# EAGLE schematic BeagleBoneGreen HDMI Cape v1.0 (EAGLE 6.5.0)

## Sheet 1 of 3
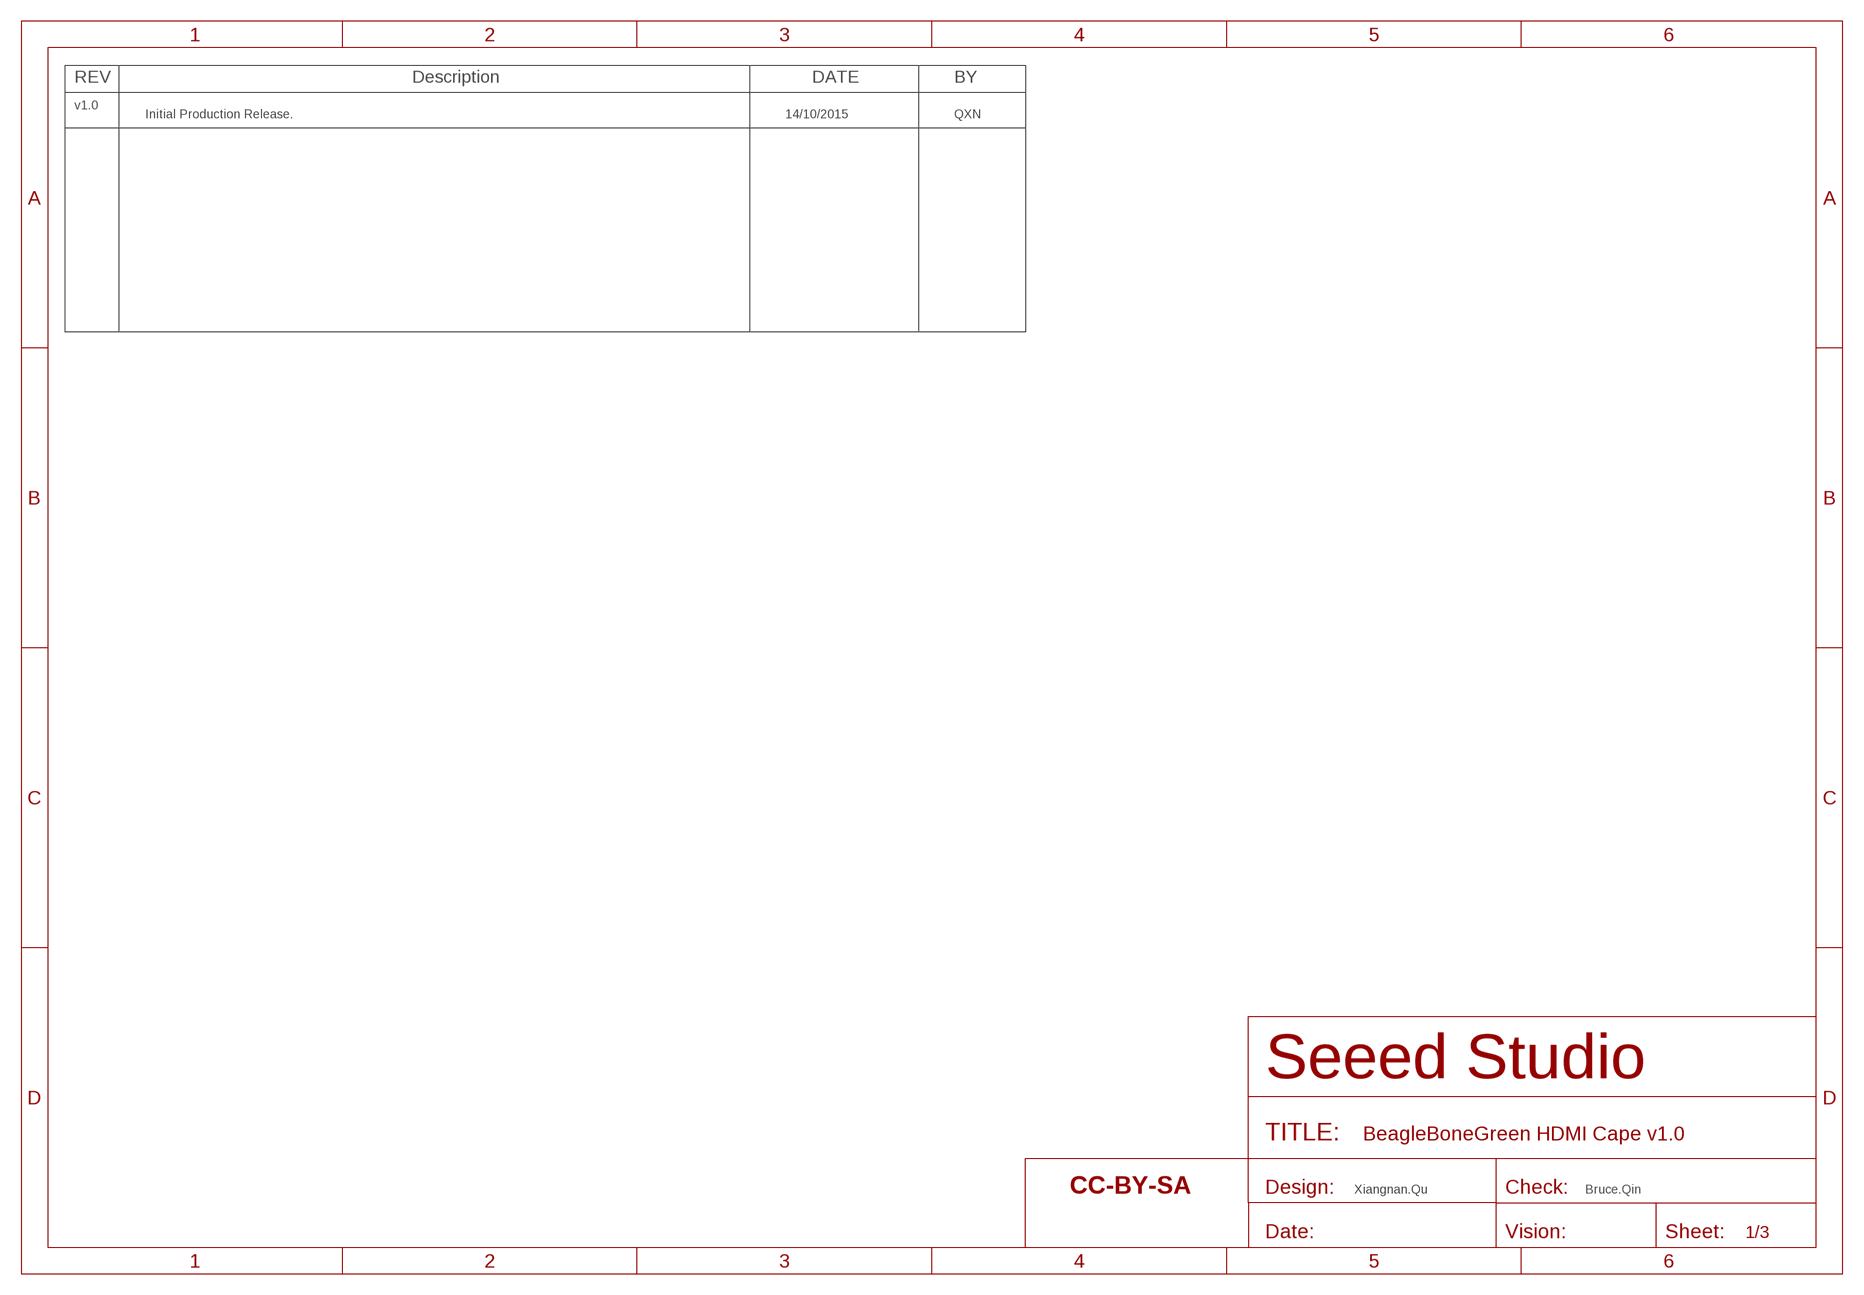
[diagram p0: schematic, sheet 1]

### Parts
FR1  SEEEDSTUDIO-OPEN-SCH-FRAME  [SEEEDSTUDIO-PCB-FRAME]

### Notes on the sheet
- REV | Description | DATE | BY
- v1.0
- Initial Production Release. | 14/10/2015 | QXN
- Xiangnan.Qu | Bruce.Qin

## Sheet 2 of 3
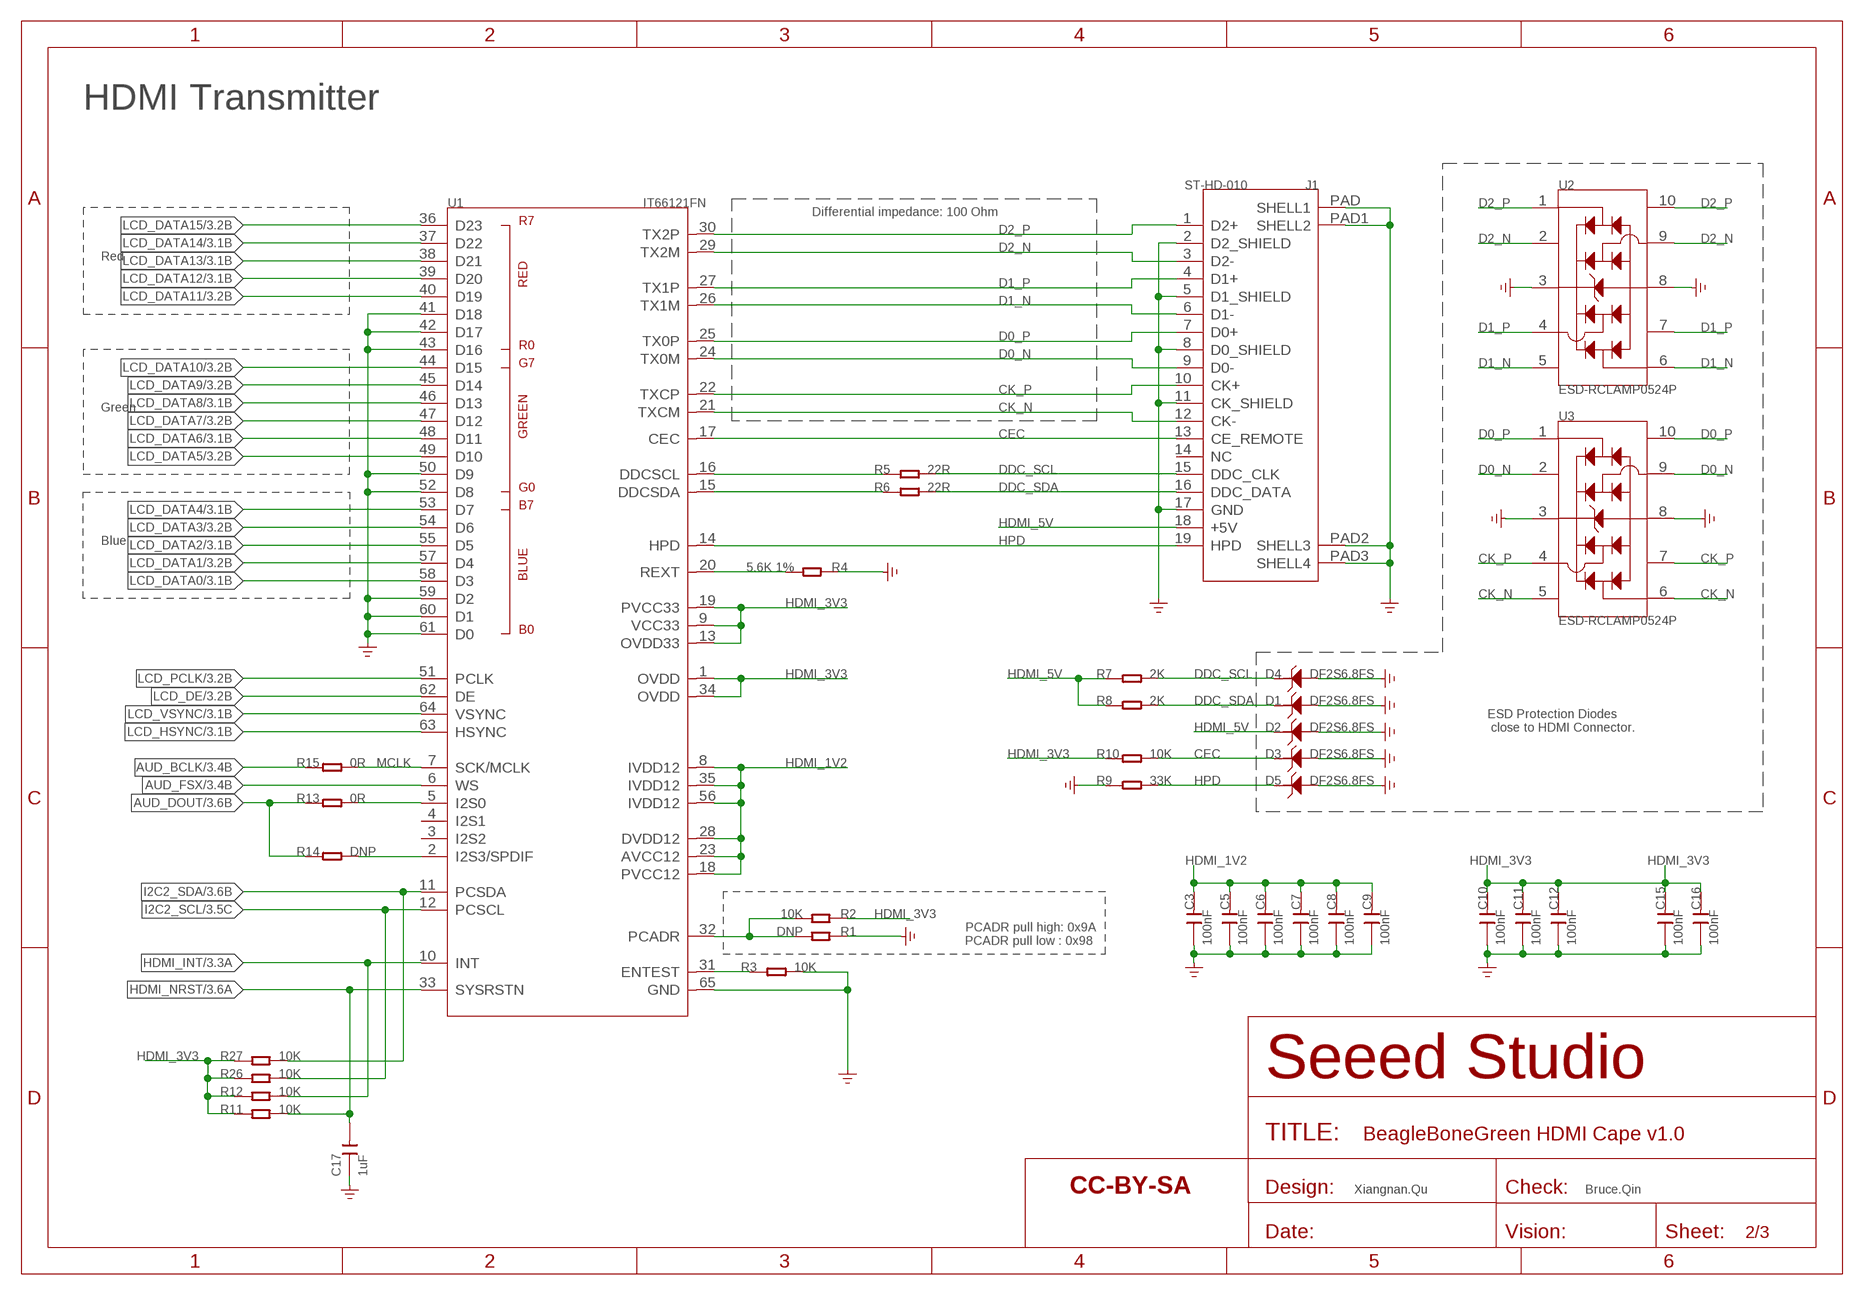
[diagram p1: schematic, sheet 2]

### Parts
C3  100nF  CAP-0402  [C0402]
C5  100nF  CAP-0402  [C0402]
C6  100nF  CAP-0402  [C0402]
C7  100nF  CAP-0402  [C0402]
C8  100nF  CAP-0402  [C0402]
C9  100nF  CAP-0402  [C0402]
C10  100nF  CAP-0402  [C0402]
C11  100nF  CAP-0402  [C0402]
C12  100nF  CAP-0402  [C0402]
C15  100nF  CAP-0402  [C0402]
C16  100nF  CAP-0402  [C0402]
C17  1uF  CAP-0603  [C0603]
D1  DF2S6.8FS  D-ESD-2P'DF2S6.8FS'  [SOD-923]
D2  DF2S6.8FS  D-ESD-2P'DF2S6.8FS'  [SOD-923]
D3  DF2S6.8FS  D-ESD-2P'DF2S6.8FS'  [SOD-923]
D4  DF2S6.8FS  D-ESD-2P'DF2S6.8FS'  [SOD-923]
D5  DF2S6.8FS  D-ESD-2P'DF2S6.8FS'  [SOD-923]
FR2  SEEEDSTUDIO-OPEN-SCH-FRAME  [SEEEDSTUDIO-PCB-FRAME]
J1  ST-HD-010  CONNECTOR-HDMI-19P  [HDMI19P-0.5-15X12.15X6.18MM]
R1  DNP  RES-0402  [R0402]
R2  10K  RES-0402  [R0402]
R3  10K  RES-0402  [R0402]
R4  5.6K 1%  RES-0402  [R0402]
R5  22R  RES-0402  [R0402]
R6  22R  RES-0402  [R0402]
R7  2K  RES-0402  [R0402]
R8  2K  RES-0402  [R0402]
R9  33K  RES-0402  [R0402]
R10  10K  RES-0402  [R0402]
R11  10K  RES-0402  [R0402]
R12  10K  RES-0402  [R0402]
R13  0R  RES-0402  [R0402]
R14  DNP  RES-0402  [R0402]
R15  0R  RES-0402  [R0402]
R26  10K  RES-0402  [R0402]
R27  10K  RES-0402  [R0402]
U1  IT66121FN  TRANSFER_IT66121FN-9  [QFN64-0.5-9X9MM]
U2  ESD-RCLAMP0524P  [ESD10P-0.5-2.5X1X0.58MM]
U3  ESD-RCLAMP0524P  [ESD10P-0.5-2.5X1X0.58MM]

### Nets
AUD_BCLK: R15.1 ; also sheet 3
AUD_DOUT: R13.1 R14.1 ; also sheet 3
AUD_FSX: U1.6(WS) ; also sheet 3
CEC: D3.1 J1.13(CE_REMOTE) R10.2 U1.17(CEC)
CK_N: J1.12(CK-) U1.21(TXCM) U3.5 U3.6
CK_P: J1.10(CK+) U1.22(TXCP) U3.4 U3.7
D0_N: J1.9(D0-) U1.24(TX0M) U3.2 U3.9
D0_P: J1.7(D0+) U1.25(TX0P) U3.1 U3.10
D1_N: J1.6(D1-) U1.26(TX1M) U2.5 U2.6
D1_P: J1.4(D1+) U1.27(TX1P) U2.4 U2.7
D2_N: J1.3(D2-) U1.29(TX2M) U2.2 U2.9
D2_P: J1.1(D2+) U1.30(TX2P) U2.1 U2.10
DDC_SCL: D4.1 J1.15(DDC_CLK) R5.2 R7.2
DDC_SDA: D1.1 J1.16(DDC_DATA) R6.2 R8.2
GND: C3.1 C5.1 C6.1 C7.1 C8.1 C9.1 C10.1 C11.1 C12.1 C15.1 C16.1 C17.1 D1.2 D2.2 D3.2 D4.2 D5.2 J1.2(D2_SHIELD) J1.5(D1_SHIELD) J1.8(D0_SHIELD) J1.11(CK_SHIELD) J1.17(GND) J1.PAD1(SHELL2) J1.PAD2(SHELL3) J1.PAD3(SHELL4) J1.PAD(SHELL1) R1.1 R3.2 R4.1 R9.1 U1.41(D18) U1.42(D17) U1.43(D16) U1.50(D9) U1.52(D8) U1.59(D2) U1.60(D1) U1.61(D0) U1.65(GND) U2.3 U2.8 U3.3 U3.8 ; supply symbol labelled GND_POWER ; also sheet 3
HDMI_1V2: C3.2 C5.2 C6.2 C7.2 C8.2 C9.2 U1.8(IVDD12) U1.18(PVCC12) U1.23(AVCC12) U1.28(DVDD12) U1.35(IVDD12) U1.56(IVDD12) ; also sheet 3
HDMI_3V3: C10.2 C11.2 C12.2 C15.2 C16.2 R2.1 R10.1 R11.1 R12.1 R26.1 R27.1 U1.1(OVDD) U1.9(VCC33) U1.13(OVDD33) U1.19(PVCC33) U1.34(OVDD) ; also sheet 3
HDMI_5V: D2.1 J1.18(+5V) R7.1 R8.1 ; also sheet 3
HDMI_INT: R12.2 U1.10(INT) ; also sheet 3
HDMI_NRST: C17.2 R11.2 U1.33(SYSRSTN) ; also sheet 3
HPD: D5.1 J1.19(HPD) R9.2 U1.14(HPD)
I2C2_SCL: R26.2 U1.12(PCSCL) ; also sheet 3
I2C2_SDA: R27.2 U1.11(PCSDA) ; also sheet 3
LCD_DATA0: U1.58(D3) ; also sheet 3
LCD_DATA1: U1.57(D4) ; also sheet 3
LCD_DATA2: U1.55(D5) ; also sheet 3
LCD_DATA3: U1.54(D6) ; also sheet 3
LCD_DATA4: U1.53(D7) ; also sheet 3
LCD_DATA5: U1.49(D10) ; also sheet 3
LCD_DATA6: U1.48(D11) ; also sheet 3
LCD_DATA7: U1.47(D12) ; also sheet 3
LCD_DATA8: U1.46(D13) ; also sheet 3
LCD_DATA9: U1.45(D14) ; also sheet 3
LCD_DATA10: U1.44(D15) ; also sheet 3
LCD_DATA11: U1.40(D19) ; also sheet 3
LCD_DATA12: U1.39(D20) ; also sheet 3
LCD_DATA13: U1.38(D21) ; also sheet 3
LCD_DATA14: U1.37(D22) ; also sheet 3
LCD_DATA15: U1.36(D23) ; also sheet 3
LCD_DE: U1.62(DE) ; also sheet 3
LCD_HSYNC: U1.63(HSYNC) ; also sheet 3
LCD_PCLK: U1.51(PCLK) ; also sheet 3
LCD_VSYNC: U1.64(VSYNC) ; also sheet 3
MCLK: R15.2 U1.7(SCK/MCLK) ; also sheet 3
N$3: R14.2 U1.2(I2S3/SPDIF)
N$4: R13.2 U1.5(I2S0)
N$8: R1.2 R2.2 U1.32(PCADR)
N$34: R3.1 U1.31(ENTEST)
N$44: R4.2 U1.20(REXT)
N$83: R5.1 U1.16(DDCSCL)
N$85: R6.1 U1.15(DDCSDA)
Unconnected: J1.14(NC) U1.3(I2S2) U1.4(I2S1)

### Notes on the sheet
- HDMI Transmitter
- Differential impedance: 100 Ohm
- Red
- Green
- Blue
- ESD Protection Diodes 
   close to HDMI Connector.
- PCADR pull high: 0x9A
  PCADR pull low : 0x98
- Xiangnan.Qu | Bruce.Qin

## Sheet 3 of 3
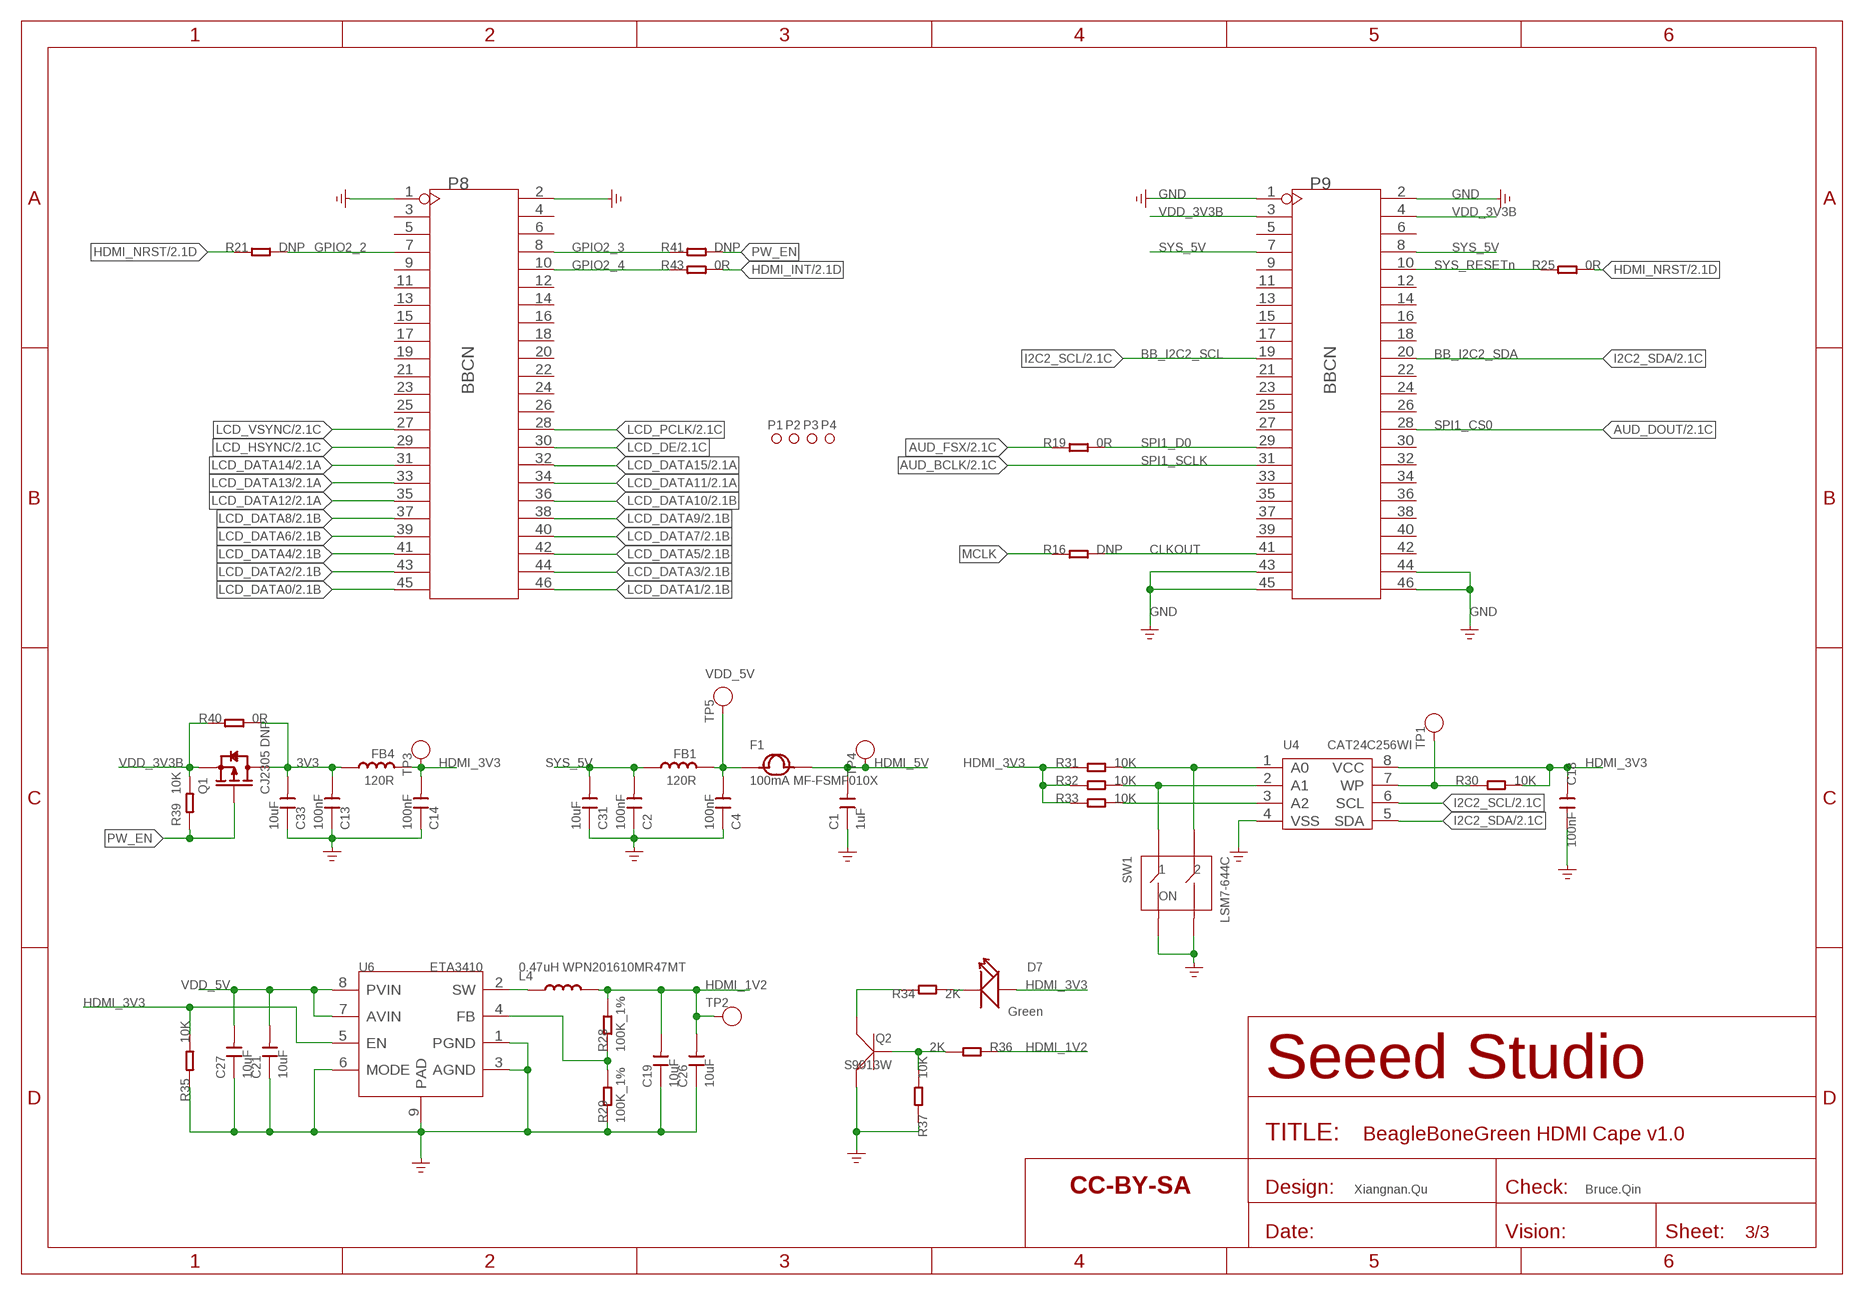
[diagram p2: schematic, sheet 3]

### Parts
C1  1uF  CAP-0603  [C0603]
C2  100nF  CAP-0603  [C0603]
C4  100nF  CAP-0603  [C0603]
C13  100nF  CAP-0603  [C0603]
C14  100nF  CAP-0603  [C0603]
C18  100nF  CAP-0402  [C0402]
C19  10uF  CAP-0603  [C0603]
C21  10uF  CAP-0603  [C0603]
C26  10uF  CAP-0603  [C0603]
C27  10uF  CAP-0603  [C0603]
C31  10uF  CAP-0603  [C0603]
C33  10uF  CAP-0603  [C0603]
D7  Green  LED'0805'  [LED-0805]
F1  100mA MF-FSMF010X  FUSE0603  [F0603]
FB1  120R  INDUCTOR/FERRITE-BEAD'0603'  [L0603]
FB4  120R  INDUCTOR/FERRITE-BEAD'0603'  [L0603]
FR4  SEEEDSTUDIO-OPEN-SCH-FRAME  [SEEEDSTUDIO-PCB-FRAME]
L4  0.47uH WPN201610MR47MT  L-MPM201610SR33_T  [L201610]
P1  MARK-1.0'ANNULAR'  [ROUND-MARK-1.0]
P2  MARK-1.0'ANNULAR'  [ROUND-MARK-1.0]
P3  MARK-1.0'ANNULAR'  [ROUND-MARK-1.0]
P4  MARK-1.0'ANNULAR'  [ROUND-MARK-1.0]
P8  BBCN  HEADER-2X23P  [2X23P-2.54]
P9  BBCN  HEADER-2X23P  [2X23P-2.54]
Q1  CJ2305 DNP  MOSFET-P'SI2323CDS/SI2305DS<BR>'  [SOT-23]
Q2  S9013W  TRANSISTOR-NPN-SOT323  [SOT-323]
R16  DNP  RES-0402  [R0402]
R19  0R  RES-0402  [R0402]
R21  DNP  RES-0402  [R0402]
R25  0R  RES-0402  [R0402]
R28  100K_1%  RES-0402  [R0402]
R29  100K_1%  RES-0402  [R0402]
R30  10K  RES-0402  [R0402]
R31  10K  RES-0402  [R0402]
R32  10K  RES-0402  [R0402]
R33  10K  RES-0402  [R0402]
R34  2K  RES-0402  [R0402]
R35  10K  RES-0402  [R0402]
R36  2K  RES-0402  [R0402]
R37  10K  RES-0402  [R0402]
R39  10K  RES-0402  [R0402]
R40  0R  RES-0603  [R0603]
R41  DNP  RES-0402  [R0402]
R43  0R  RES-0402  [R0402]
SW1  LSM7-644C  SWITCHES-4P'KM-02'  [SW4-SMD-5.08X6.8X3.3MM]
TP1  TEST-POINT  [TP-D65/35MIL]
TP2  TEST-POINT  [TP-D65/35MIL]
TP3  TEST-POINT  [TP-D65/35MIL]
TP4  TEST-POINT  [TP-D65/35MIL]
TP5  TEST-POINT  [TP-D65/35MIL]
U4  CAT24C256WI  MCU-EEPROM-CAT24C256  [SOIC8-1.27-5X4MM]
U6  ETA3410  CONVERTER-ETA3410  [DFN8G-0.5-2X2MM]

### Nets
3V3: C13.2 C33.2 FB4.2 Q1.3(D) R40.2
AUD_BCLK: P9.31 ; also sheet 2
AUD_DOUT: P9.28 ; also sheet 2
AUD_FSX: R19.1 ; also sheet 2
CLKOUT: P9.41 R16.2
GND: C1.1 C2.1 C4.1 C13.1 C14.1 C18.1 C19.1 C21.1 C26.1 C27.1 C31.1 C33.1 P8.1 P8.2 P9.1 P9.2 P9.43 P9.44 P9.45 P9.46 Q2.2(E) R29.1 R35.1 R37.2 SW1.3 SW1.4 U4.4(VSS) U6.1(PGND) U6.3(AGND) U6.6(MODE) U6.9(PAD) ; supply symbol labelled GND_POWER ; also sheet 2
HDMI_1V2: C19.2 C26.2 L4.2 R28.2 R36.2 TP2.P1(T) ; also sheet 2
HDMI_3V3: C14.2 C18.2 D7.+ FB4.1 R30.1 R31.2 R32.2 R33.2 R35.2 TP3.P1(T) U4.8(VCC) U6.5(EN) ; also sheet 2
HDMI_5V: C1.2 F1.2 TP4.P1(T) ; also sheet 2
HDMI_INT: R43.2 ; also sheet 2
HDMI_NRST: R21.1 R25.2 ; also sheet 2
I2C2_SCL: P9.19 U4.6(SCL) ; also sheet 2
I2C2_SDA: P9.20 U4.5(SDA) ; also sheet 2
LCD_DATA0: P8.45 ; also sheet 2
LCD_DATA1: P8.46 ; also sheet 2
LCD_DATA2: P8.43 ; also sheet 2
LCD_DATA3: P8.44 ; also sheet 2
LCD_DATA4: P8.41 ; also sheet 2
LCD_DATA5: P8.42 ; also sheet 2
LCD_DATA6: P8.39 ; also sheet 2
LCD_DATA7: P8.40 ; also sheet 2
LCD_DATA8: P8.37 ; also sheet 2
LCD_DATA9: P8.38 ; also sheet 2
LCD_DATA10: P8.36 ; also sheet 2
LCD_DATA11: P8.34 ; also sheet 2
LCD_DATA12: P8.35 ; also sheet 2
LCD_DATA13: P8.33 ; also sheet 2
LCD_DATA14: P8.31 ; also sheet 2
LCD_DATA15: P8.32 ; also sheet 2
LCD_DE: P8.30 ; also sheet 2
LCD_HSYNC: P8.29 ; also sheet 2
LCD_PCLK: P8.28 ; also sheet 2
LCD_VSYNC: P8.27 ; also sheet 2
MCLK: R16.1 ; also sheet 2
N$1: P8.7 R21.2
N$2: P8.8 R41.1
N$6: Q2.1(B) R36.1 R37.1
N$9: P9.29 R19.2
N$12: R30.2 TP1.P1(T) U4.7(WP)
N$13: R31.1 SW1.2 U4.1(A0)
N$16: R32.1 SW1.1 U4.2(A1)
N$17: R33.1 U4.3(A2)
N$18: P9.10 R25.1
N$19: Q2.3(C) R34.1
N$21: D7.- R34.2
N$23: P8.10 R43.1
N$75: L4.1 U6.2(SW)
N$76: R28.1 R29.2 U6.4(FB)
PW_EN: Q1.1(G) R39.2 R41.2
SYS_5V: C2.2 C31.2 FB1.2 P9.7 P9.8
VDD_3V3B: P9.3 P9.4 Q1.2(S) R39.1 R40.1
VDD_5V: C4.2 C21.2 C27.2 F1.1 FB1.1 TP5.P1(T) U6.7(AVIN) U6.8(PVIN)
Unconnected: P8.3 P8.4 P8.5 P8.6 P8.9 P8.11 P8.12 P8.13 P8.14 P8.15 P8.16 P8.17 P8.18 P8.19 P8.20 P8.21 P8.22 P8.23 P8.24 P8.25 P8.26 P9.5 P9.6 P9.9 P9.11 P9.12 P9.13 P9.14 P9.15 P9.16 P9.17 P9.18 P9.21 P9.22 P9.23 P9.24 P9.25 P9.26 P9.27 P9.30 P9.32 P9.33 P9.34 P9.35 P9.36 P9.37 P9.38 P9.39 P9.40 P9.42

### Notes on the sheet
- GPIO2_2 | GPIO2_3
- GPIO2_4 | SYS_RESETn
- BB_I2C2_SCL | BB_I2C2_SDA
- SPI1_CS0
- SPI1_D0
- SPI1_SCLK
- Xiangnan.Qu | Bruce.Qin

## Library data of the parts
C1-C19 C21 C26 C27 C31 C33 = Discrete-new:CAP: Ceramic Capacitors
D1-D5 = Discrete-new:D-ESD-2P: SOD-923:304060009;SOD-123:304060001
D7 = Discrete-new:LED
F1 = Discrete-new:FUSE
FB1 FB4 = Discrete-new:INDUCTOR/FERRITE-BEAD
FR1 FR2 FR4 = moudle-new:SEEEDSTUDIO-OPEN-SCH-FRAME
J1 = template:CONNECTOR-HDMI-19P
L4 = Discrete-new:L
P1-P4 = Discrete-new:MARK-1.0; PARTNO: DNP
P8 P9 = Connector :HEADER-2X23P
Q1 = Discrete-new:MOSFET-P
Q2 = Discrete-new:TRANSISTOR-NPN: NPN audion
R1-R16 R19 R21 R25-R37 R39-R41 R43 = Discrete-new:RES
SW1 = Discrete-new:SWITCHES-4P
TP1-TP5 = Discrete-new:TEST-POINT
U1 = template:TRANSFER_IT66121FN
U2 U3 = template:ESD-RCLAMP0524P
U4 = template:MCU-EEPROM-CAT24C256: 256 kb I2C CMOS Serial EEPROM
U6 = template:CONVERTER-ETA3410: 3MHZ 2A High Step-Down Converter in DFN2x2-8L Package

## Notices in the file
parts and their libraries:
moudle-new: This work is licensed under the Creative Commons Attribution 4.0 International License.
To view a copy of this license,visit:
http://creativecommons.org/licenses/by-sa/4.0
moudle-new: CC-BY-SA
